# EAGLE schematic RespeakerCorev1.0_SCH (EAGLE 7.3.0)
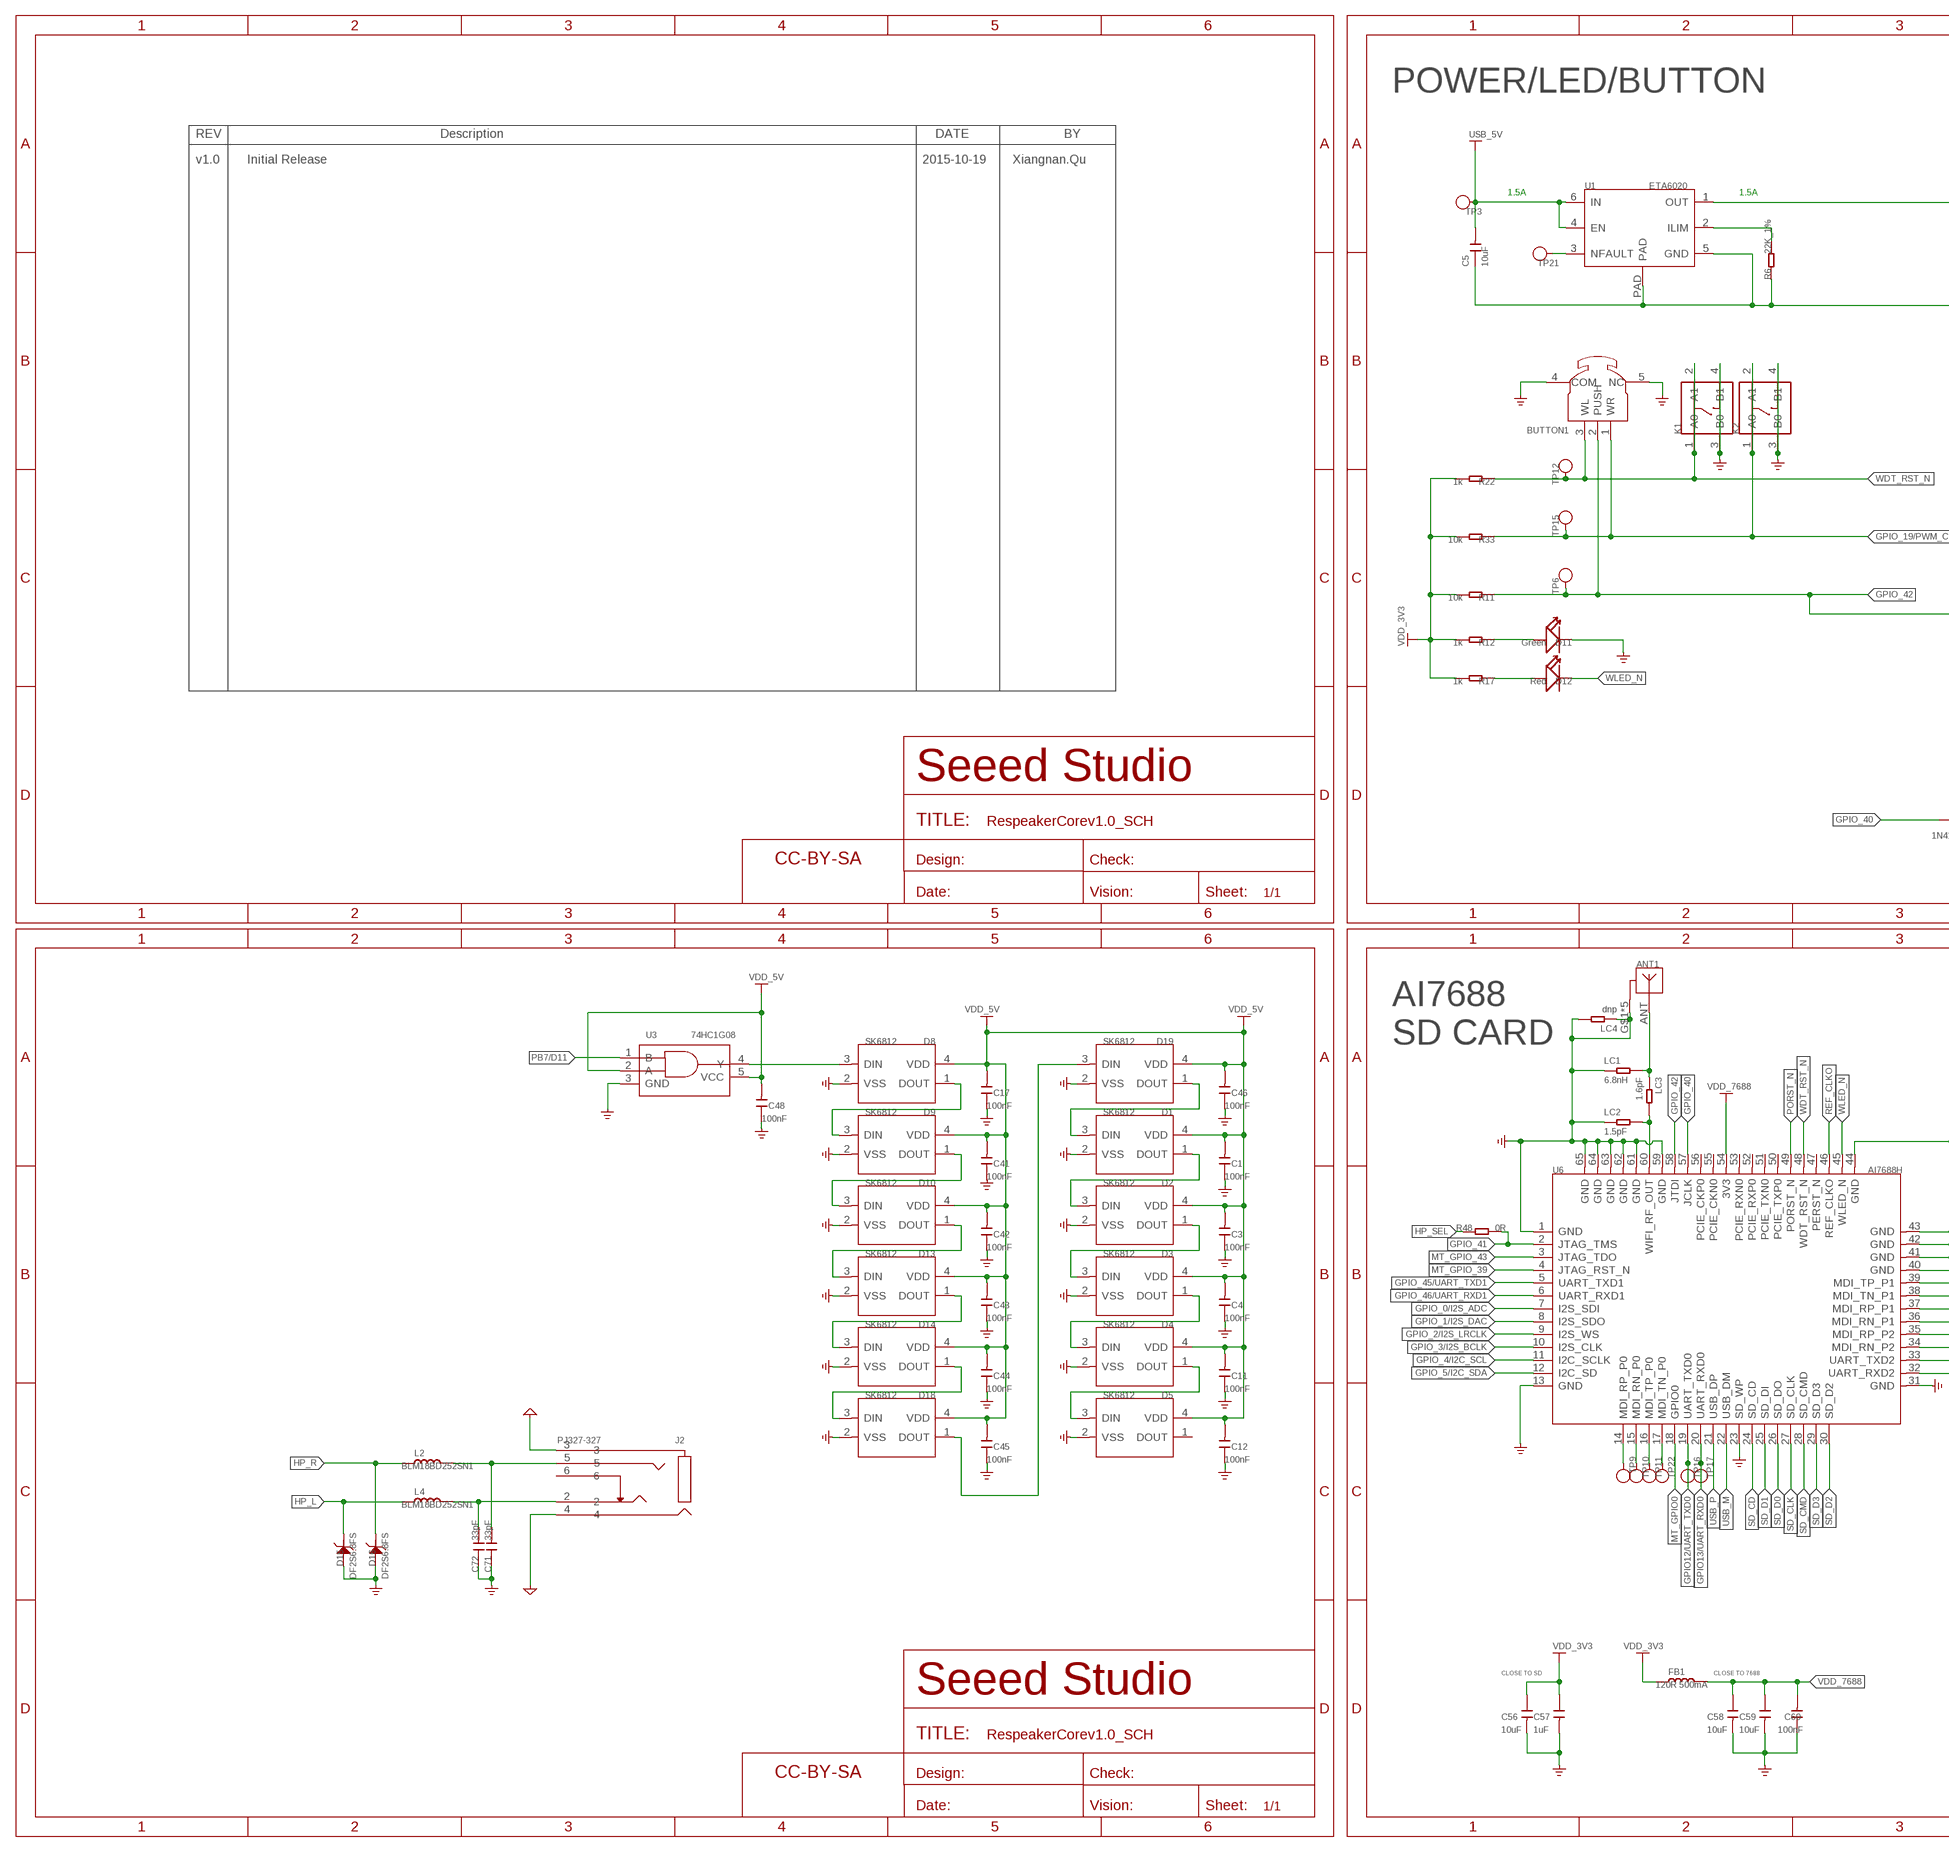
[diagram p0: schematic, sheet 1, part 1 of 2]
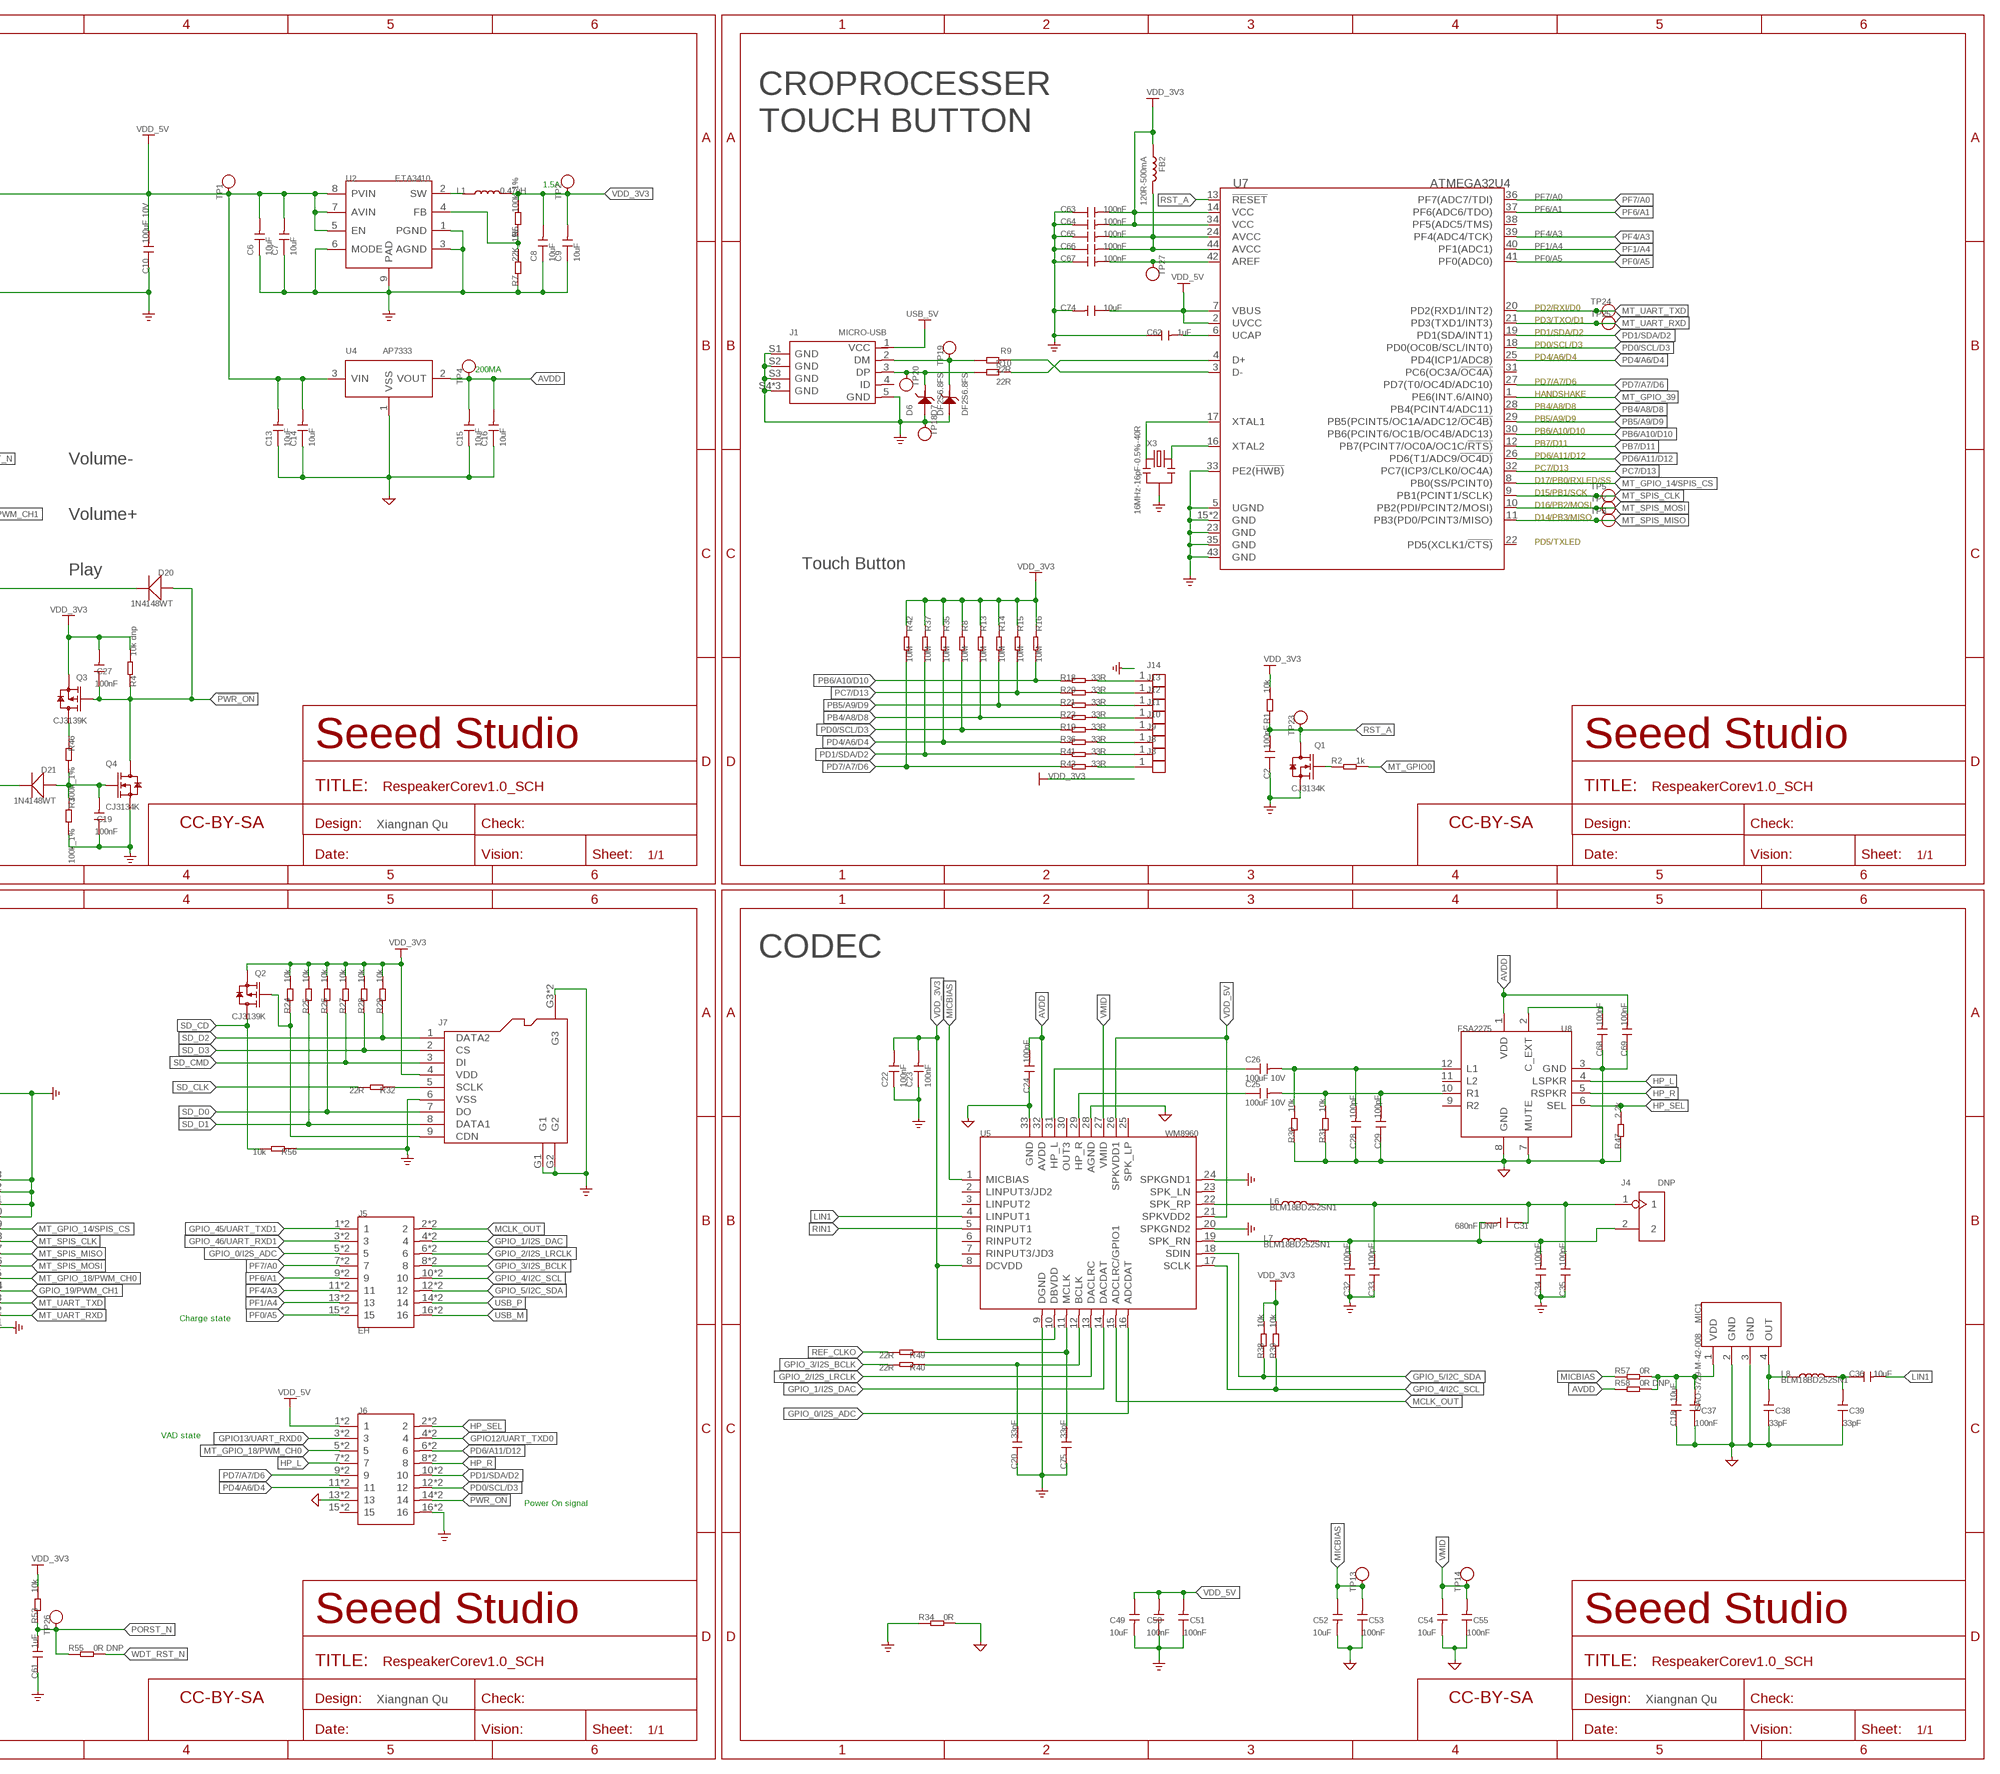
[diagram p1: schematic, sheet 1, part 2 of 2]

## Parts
ANT1  ANTENNA-ACA2012-BOTTOM  [ANT2P-SMD-3.5X1.4MM-BOTTOM]
BUTTON1  BUTTON3+2P  [BUTTON3+2P-SMD-11.8X11.8X2.5MM]
C1  100nF  CAP-0402  [C0402]
C2  100nF  CAP-0402  [C0402]
C3  100nF  CAP-0402  [C0402]
C4  100nF  CAP-0402  [C0402]
C5  10uF  CAP-0603  [C0603]
C6  10uF  CAP-0603  [C0603]
C7  10uF  CAP-0603  [C0603]
C8  10uF  CAP-0603  [C0603]
C9  10uF  CAP-0603  [C0603]
C10  100uF 10V  CAP-1206  [C1206]
C11  100nF  CAP-0402  [C0402]
C12  100nF  CAP-0402  [C0402]
C13  10uF  CAP-0603  [C0603]
C14  10uF  CAP-0603  [C0603]
C15  10uF  CAP-0603  [C0603]
C16  10uF  CAP-0603  [C0603]
C17  100nF  CAP-0402  [C0402]
C18  10uF  CAP-0603  [C0603]
C19  100nF  CAP-0402  [C0402]
C20  33pF  CAP-0402  [C0402]
C22  100nF  CAP-0402  [C0402]
C23  100nF  CAP-0402  [C0402]
C24  100nF  CAP-0402  [C0402]
C25  100uF 10V  CAP-1206  [C1206]
C26  100uF 10V  CAP-1206  [C1206]
C27  100nF  CAP-0402  [C0402]
C28  100pF  CAP-0402  [C0402]
C29  100pF  CAP-0402  [C0402]
C31  680nF DNP  CAP-0402  [C0402]
C32  100pF  CAP-0402  [C0402]
C33  100pF  CAP-0402  [C0402]
C34  100pF  CAP-0402  [C0402]
C35  100pF  CAP-0402  [C0402]
C36  10uF  CAP-0603  [C0603]
C37  100nF  CAP-0402  [C0402]
C38  33pF  CAP-0402  [C0402]
C39  33pF  CAP-0402  [C0402]
C41  100nF  CAP-0402  [C0402]
C42  100nF  CAP-0402  [C0402]
C43  100nF  CAP-0402  [C0402]
C44  100nF  CAP-0402  [C0402]
C45  100nF  CAP-0402  [C0402]
C46  100nF  CAP-0402  [C0402]
C48  100nF  CAP-0402  [C0402]
C49  10uF  CAP-0603  [C0603]
C50  100nF  CAP-0402  [C0402]
C51  100nF  CAP-0402  [C0402]
C52  10uF  CAP-0603  [C0603]
C53  100nF  CAP-0402  [C0402]
C54  10uF  CAP-0603  [C0603]
C55  100nF  CAP-0402  [C0402]
C56  10uF  CAP-0603  [C0603]
C57  1uF  CAP-0402  [C0402]
C58  10uF  CAP-0603  [C0603]
C59  10uF  CAP-0603  [C0603]
C60  100nF  CAP-0402  [C0402]
C61  1uF  CAP-0402  [C0402]
C62  1uF  CAP-0402  [C0402]
C63  100nF  CAP-0402  [C0402]
C64  100nF  CAP-0402  [C0402]
C65  100nF  CAP-0402  [C0402]
C66  100nF  CAP-0402  [C0402]
C67  100nF  CAP-0402  [C0402]
C68  100nF  CAP-0402  [C0402]
C69  100nF  CAP-0402  [C0402]
C71  33pF  CAP-0402  [C0402]
C72  33pF  CAP-0402  [C0402]
C74  10uF  CAP-0603  [C0603]
C75  33pF  CAP-0402  [C0402]
D1  SK6812  LED-RGB-4P-SK68122  [LED4-SMD-3.5X3.7MM]
D2  SK6812  LED-RGB-4P-SK68122  [LED4-SMD-3.5X3.7MM]
D3  SK6812  LED-RGB-4P-SK68122  [LED4-SMD-3.5X3.7MM]
D4  SK6812  LED-RGB-4P-SK68122  [LED4-SMD-3.5X3.7MM]
D5  SK6812  LED-RGB-4P-SK68122  [LED4-SMD-3.5X3.7MM]
D6  DF2S6.8FS  D-ESD-2P'DF2S6.8FS'  [SOD-923]
D7  DF2S6.8FS  D-ESD-2P'DF2S6.8FS'  [SOD-923]
D8  SK6812  LED-RGB-4P-SK68122  [LED4-SMD-3.5X3.7MM]
D9  SK6812  LED-RGB-4P-SK68122  [LED4-SMD-3.5X3.7MM]
D10  SK6812  LED-RGB-4P-SK68122  [LED4-SMD-3.5X3.7MM]
D11  Green  LED'RIGHT'  [LED-SIDE-VIEW-0603-RIGHT]
D12  Red  LED'RIGHT'  [LED-SIDE-VIEW-0603-RIGHT]
D13  SK6812  LED-RGB-4P-SK68122  [LED4-SMD-3.5X3.7MM]
D14  SK6812  LED-RGB-4P-SK68122  [LED4-SMD-3.5X3.7MM]
D15  DF2S6.8FS  D-ESD-2P'DF2S6.8FS'  [SOD-923]
D16  DF2S6.8FS  D-ESD-2P'DF2S6.8FS'  [SOD-923]
D18  SK6812  LED-RGB-4P-SK68122  [LED4-SMD-3.5X3.7MM]
D19  SK6812  LED-RGB-4P-SK68122  [LED4-SMD-3.5X3.7MM]
D20  1N4148WT  DIODE'0603'  [SOD-523]
D21  1N4148WT  DIODE'0603'  [SOD-523]
FB1  120R 500mA  INDUCTOR/FERRITE-BEAD'0603'  [L0603]
FB2  120R-500mA  INDUCTOR/FERRITE-BEAD'0603'  [L0603]
FR1  SEEEDSTUDIO-OPEN-SCH-FRAME  [SEEEDSTUDIO-PCB-FRAME]
FR2  SEEEDSTUDIO-OPEN-SCH-FRAME  [SEEEDSTUDIO-PCB-FRAME]
FR3  SEEEDSTUDIO-OPEN-SCH-FRAME  [SEEEDSTUDIO-PCB-FRAME]
FR4  SEEEDSTUDIO-OPEN-SCH-FRAME  [SEEEDSTUDIO-PCB-FRAME]
FR5  SEEEDSTUDIO-OPEN-SCH-FRAME  [SEEEDSTUDIO-PCB-FRAME]
FR7  SEEEDSTUDIO-OPEN-SCH-FRAME  [SEEEDSTUDIO-PCB-FRAME]
J1  MICRO-USB  MICRO-USB5+4P'5+4P'  [MICRO-USB5+4P-SMD-0.65-B]
J2  PJ327-327  AUDIO-JACK-5P-PJ327-327  [AUDIO5P-14X5X4.4MM]
J3  HEADER-1P-3MM  [1P-DIP-6X4MM]
J4  DNP  HEADER-2P-65/35MIL  [H2-2.54]
J5  EH  HEADER-2X8P-SMD_DRILL-2.0  [H2X8-SMD_DRILL-2.0]
J6  HEADER-2X8P-SMD_DRILL-2.0  [H2X8-SMD_DRILL-2.0]
J7  MICRO-SD-CARD-HOLDER-9P'MICROSD-9P'  [MICRO-SD9+4P-SMD-16.1X14.5X1.85MM]
J8  HEADER-1P-3MM  [1P-DIP-6X4MM]
J9  HEADER-1P-3MM  [1P-DIP-6X4MM]
J10  HEADER-1P-3MM  [1P-DIP-6X4MM]
J11  HEADER-1P-3MM  [1P-DIP-6X4MM]
J12  HEADER-1P-3MM  [1P-DIP-6X4MM]
J13  HEADER-1P-3MM  [1P-DIP-6X4MM]
J14  HEADER-1P-3MM  [1P-DIP-6X4MM]
K1  BUTTON-4P-4.5X3.2  [SW4P-SMD-4.5X3.2X2.5MM]
K2  BUTTON-4P-4.5X3.2  [SW4P-SMD-4.5X3.2X2.5MM]
L1  0.47uH  L-MPM201610SR33_T  [L201610]
L2  BLM18BD252SN1  INDUCTOR/FERRITE-BEAD'0603'  [L0603]
L4  BLM18BD252SN1  INDUCTOR/FERRITE-BEAD'0603'  [L0603]
L6  BLM18BD252SN1  INDUCTOR/FERRITE-BEAD'0603'  [L0603]
L7  BLM18BD252SN1  INDUCTOR/FERRITE-BEAD'0603'  [L0603]
L8  BLM18BD252SN1  INDUCTOR/FERRITE-BEAD'0603'  [L0603]
LC1  6.8nH  RES-0402  [R0402]
LC2  1.5pF  RES-0402  [R0402]
LC3  1.6pF  RES-0402  [R0402]
LC4  dnp  RES-0402  [R0402]
MIC1  SAO-3729-M-42-008  MIC-MSM421A3729H8-C  [MIC4-SMD-3.76X2.95MM]
Q1  CJ3134K  MOSFET-N-CJ3134K  [SOT-723]
Q2  CJ3139K  MOSFET-P-CJ3139K  [SOT-723]
Q3  CJ3139K  MOSFET-P-CJ3139K  [SOT-723]
Q4  CJ3134K  MOSFET-N-CJ3134K  [SOT-723]
R1  10k  RES-0402  [R0402]
R2  1k  RES-0402  [R0402]
R3  100k_1%  RES-0402  [R0402]
R4  10k dnp  RES-0402  [R0402]
R5  100k_1%  RES-0402  [R0402]
R6  22K_1%  RES-0402  [R0402]
R7  22K_1%  RES-0402  [R0402]
R8  10M  RES-0402  [R0402]
R9  22R  RES-0402  [R0402]
R10  22R  RES-0402  [R0402]
R11  10k  RES-0402  [R0402]
R12  1k  RES-0402  [R0402]
R13  10M  RES-0402  [R0402]
R14  10M  RES-0402  [R0402]
R15  10M  RES-0402  [R0402]
R16  10M  RES-0402  [R0402]
R17  1k  RES-0402  [R0402]
R18  33R  RES-0402  [R0402]
R19  33R  RES-0402  [R0402]
R20  33R  RES-0402  [R0402]
R21  33R  RES-0402  [R0402]
R22  1k  RES-0402  [R0402]
R23  33R  RES-0402  [R0402]
R24  10k  RES-0402  [R0402]
R25  10k  RES-0402  [R0402]
R26  10k  RES-0402  [R0402]
R27  10k  RES-0402  [R0402]
R28  10k  RES-0402  [R0402]
R29  10k  RES-0402  [R0402]
R30  10k  RES-0402  [R0402]
R31  10k  RES-0402  [R0402]
R32  22R  RES-0402  [R0402]
R33  10k  RES-0402  [R0402]
R34  0R  RES-0402  [R0402]
R35  10M  RES-0402  [R0402]
R36  33R  RES-0402  [R0402]
R37  10M  RES-0402  [R0402]
R38  10k  RES-0402  [R0402]
R39  10k  RES-0402  [R0402]
R40  22R  RES-0402  [R0402]
R41  33R  RES-0402  [R0402]
R42  10M  RES-0402  [R0402]
R43  33R  RES-0402  [R0402]
R46  100k_1%  RES-0402  [R0402]
R47  2.2k  RES-0402  [R0402]
R48  0R  RES-0402  [R0402]
R49  22R  RES-0402  [R0402]
R53  10k  RES-0402  [R0402]
R55  0R DNP  RES-0402  [R0402]
R56  10k  RES-0402  [R0402]
R57  0R  RES-0402  [R0402]
R58  0R DNP  RES-0402  [R0402]
TP1  TEST-POINT'4545'  [TP-D45MIL]
TP2  TEST-POINT'4545'  [TP-D45MIL]
TP3  TEST-POINT'4545'  [TP-D45MIL]
TP4  TEST-POINT'4545'  [TP-D45MIL]
TP5  TEST-POINT'4545'  [TP-D45MIL]
TP6  TEST-POINT'4545'  [TP-D45MIL]
TP7  TEST-POINT'4545'  [TP-D45MIL]
TP8  TEST-POINT'4545'  [TP-D45MIL]
TP9  TEST-POINT'4080'  [TP-80X40MIL]
TP10  TEST-POINT'4080'  [TP-80X40MIL]
TP11  TEST-POINT'4080'  [TP-80X40MIL]
TP12  TEST-POINT'4545'  [TP-D45MIL]
TP13  TEST-POINT'4545'  [TP-D45MIL]
TP14  TEST-POINT'4545'  [TP-D45MIL]
TP15  TEST-POINT'4545'  [TP-D45MIL]
TP16  TEST-POINT'4545'  [TP-D45MIL]
TP17  TEST-POINT'4545'  [TP-D45MIL]
TP18  TEST-POINT'4545'  [TP-D45MIL]
TP19  TEST-POINT'4545'  [TP-D45MIL]
TP20  TEST-POINT'4545'  [TP-D45MIL]
TP21  TEST-POINT'4545'  [TP-D45MIL]
TP22  TEST-POINT'4080'  [TP-80X40MIL]
TP23  TEST-POINT'4545'  [TP-D45MIL]
TP24  TEST-POINT'4545'  [TP-D45MIL]
TP25  TEST-POINT'4545'  [TP-D45MIL]
TP26  TEST-POINT'4545'  [TP-D45MIL]
TP27  TEST-POINT'4545'  [TP-D45MIL]
U1  ETA6020  PMIC-ETA6020D2G-T_UDFN6  [DFN6G-0.65-2X2MM]
U2  ETA3410  CONVERTER-ETA3410  [DFN8G-0.5-2X2MM]
U3  74HC1G08  LOGIC-74HC1G08'GW'  [SOT-353]
U4  AP7333  PMIC-XC6206PMR  [SOT-23]
U5  WM8960  AMPLIFIER-WM8960  [QFN32G-0.5-5X5MM]
U6  AI7688H  MOUDLE-IOT-AI7688H  [LGA65-1.7-24X32X1.8MM]
U7  ATMEGA32U4  MCU-ATMEGA32U4-MUR  [VQFN-44]
U8  FSA2275  SWITCH-ANALOG-FSA2275  [LEAD12P-SMD-0.4-1.8X1.8X0.5MM]
X3  16MHz-16pF-0.5%-40R  CRYSTAL-RESONATOR'SMD'  [RESONATOR3-SMD-3.6X1.3X0.8MM]

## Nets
!PWR_ON: C27.1 D20.+ J6.14 J6.P$14 Q3.1(G) Q4.3(D) R4.1
AGND: C13.1 C14.1 C15.1 C16.1 C18.1 C24.1 C28.1 C29.1 C37.1 C38.1 C39.1 C52.2 C53.1 C54.2 C55.1 C68.1 C69.1 J2.3 J2.4 J6.13 J6.P$13 MIC1.2(GND) MIC1.3(GND) R30.1 R31.1 R34.2 R47.1 U4.1(VSS) U5.28(AGND) U5.33(GND) U8.3(GND) U8.7(MUTE) U8.8(GND) ; supply symbol labelled GND_SIGNAL
AVDD: C15.2 C16.2 C24.2 C69.2 R58.1 TP4.T U4.2(VOUT) U5.32(AVDD) U8.1(VDD)
GND: ANT1.G$1 ANT1.G$2 ANT1.G$4 ANT1.GND1 ANT1.GND2 BUTTON1.4(COM) BUTTON1.5(NC) C1.1 C2.1 C3.1 C4.1 C5.1 C6.1 C7.1 C8.1 C9.1 C10.1 C11.1 C12.1 C17.1 C19.1 C20.1 C22.1 C23.1 C32.1 C33.1 C34.1 C35.1 C41.1 C42.1 C43.1 C44.1 C45.1 C46.1 C48.1 C49.2 C50.1 C51.1 C56.2 C57.2 C58.2 C59.2 C60.1 C61.1 C62.1 C63.1 C64.1 C65.1 C66.1 C67.1 C71.1 C72.1 C74.2 C75.1 D1.2(VSS) D2.2(VSS) D3.2(VSS) D4.2(VSS) D5.2(VSS) D6.2 D7.2 D8.2(VSS) D9.2(VSS) D10.2(VSS) D11.2(-) D13.2(VSS) D14.2(VSS) D15.2 D16.2 D18.2(VSS) D19.2(VSS) J1.5(GND) J1.S1(GND) J1.S2(GND) J1.S3(GND) J1.S4(GND) J1.S5(GND) J1.S6(GND) J6.16 J6.P$16 J7.6(VSS) J7.G1 J7.G2 J7.G3 J7.G4(G3) K1.3(B0) K1.4(B1) K2.3(B0) K2.4(B1) LC1.1 LC2.1 LC4.1 LC4.2 Q1.2(S) Q4.2(S) R3.2 R6.1 R7.1 R34.1 R56.1 TP18.T U1.5(GND) U1.PAD U2.1(PGND) U2.3(AGND) U2.6(MODE) U2.9(PAD) U3.3(GND) U5.9(DGND) U5.20(SPKGND2) U5.24(SPKGND1) U6.1(GND) U6.13(GND) U6.23(SD_WP) U6.31(GND) U6.40(GND) U6.41(GND) U6.42(GND) U6.43(GND) U6.44(GND) U6.59(GND) U6.61(GND) U6.62(GND) U6.63(GND) U6.64(GND) U6.65(GND) U7.5(UGND) U7.15(GND) U7.23(GND) U7.33(PE2(!HWB)) U7.35(GND) U7.43(GND) U7.TAB(GND) X3.2 ; supply symbol labelled GND_POWER
GPIO12/UART_TXD0: J6.4 J6.P$4 TP16.T U6.19(UART_TXD0)
GPIO13/UART_RXD0: J6.3 J6.P$3 TP17.T U6.20(UART_RXD0)
GPIO_0/I2S_ADC: J5.5 J5.P$5 U5.16(ADCDAT) U6.7(I2S_SDI)
GPIO_1/I2S_DAC: J5.4 J5.P$4 U5.14(DACDAT) U6.8(I2S_SDO)
GPIO_2/I2S_LRCLK: J5.6 J5.P$6 U5.13(DACLRC) U6.9(I2S_WS)
GPIO_3/I2S_BCLK: J5.8 J5.P$8 R40.2 U6.10(I2S_CLK)
GPIO_4/I2C_SCL: J5.10 J5.P$10 R39.1 U5.17(SCLK) U6.11(I2C_SCLK)
GPIO_5/I2C_SDA: J5.12 J5.P$12 R38.1 U5.18(SDIN) U6.12(I2C_SD)
GPIO_19/PWM_CH1: BUTTON1.1(WR) K2.1(A0) K2.2(A1) R33.1 TP15.T U6.34(MDI_RN_P2)
GPIO_40: D21.- U6.57(JCLK)
GPIO_41: R48.1 U6.2(JTAG_TMS)
GPIO_42: BUTTON1.2(PUSH) D20.- R11.1 TP6.T U6.58(JTDI)
GPIO_45/UART_TXD1: J5.1 J5.P$1 U6.5(UART_TXD1)
GPIO_46/UART_RXD1: J5.3 J5.P$3 U6.6(UART_RXD1)
HP_L: D15.1 J6.7 J6.P$7 L4.1 U8.4(LSPKR)
HP_R: D16.1 J6.8 J6.P$8 L2.1 U8.5(RSPKR)
HP_SEL: J6.2 J6.P$2 R47.2 R48.2 U8.6(SEL)
LIN1: C36.2 U5.4(LINPUT1)
MCLK_OUT: J5.2 J5.P$2 U5.15(ADCLRC/GPIO1)
MIC_VDD: C18.2 C37.2 MIC1.1(VDD) R57.2 R58.2
MICBIAS: C52.1 C53.2 R57.1 TP13.T U5.1(MICBIAS)
MT_GPIO0: R2.2 U6.18(GPIO0)
MT_GPIO_14/SPIS_CS: U6.39(MDI_TP_P1) U7.8(PB0(SS/PCINT0))
MT_GPIO_18/PWM_CH0: J6.5 J6.P$5 U6.35(MDI_RP_P2)
MT_GPIO_39: U6.4(JTAG_RST_N) U7.1(PE6(INT.6/AIN0))
MT_GPIO_43: U6.3(JTAG_TDO)
MT_SPIS_CLK: TP5.T U6.38(MDI_TN_P1) U7.9(PB1(PCINT1/SCLK))
MT_SPIS_MISO: TP8.T U6.37(MDI_RP_P1) U7.11(PB3(PD0/PCINT3/MISO))
MT_SPIS_MOSI: TP7.T U6.36(MDI_RN_P1) U7.10(PB2(PDI/PCINT2/MOSI))
MT_UART_RXD: TP25.T U6.32(UART_RXD2) U7.21(PD3(TXD1/INT3))
MT_UART_TXD: TP24.T U6.33(UART_TXD2) U7.20(PD2(RXD1/INT2))
N$1: Q3.3(D) R46.1
N$2: LC2.2 LC3.2 U6.60(WIFI_RF_OUT)
N$3: D11.1(+) R12.1
N$4: C68.2 U8.2(C_EXT)
N$5: C75.2 R49.1 U5.11(MCLK)
N$6: C38.2 L8.1 MIC1.4(OUT)
N$7: D12.1(+) R17.1
N$8: R10.1 U7.4(D+)
N$9: J7.5(SCLK) R32.1
N$10: R9.1 U7.3(D-)
N$11: D9.1(DOUT) D10.3(DIN)
N$12: R6.2 U1.2(ILIM)
N$13: D1.3(DIN) D19.1(DOUT)
N$14: L6.1 U5.22(SPK_RP)
N$15: D7.1 J1.2(DM) R9.2 TP19.T
N$16: D6.1 J1.3(DP) R10.2 TP20.T
N$18: D10.1(DOUT) D13.3(DIN)
N$19: D8.1(DOUT) D9.3(DIN)
N$20: J13.1 R20.2
N$21: C19.2 D21.+ Q4.1(G) R3.1 R46.2
N$22: J14.1 R18.2
N$23: D13.1(DOUT) D14.3(DIN)
N$24: C36.1 C39.2 L8.2
N$25: D14.1(DOUT) D18.3(DIN)
N$26: C20.2 R40.1 U5.12(BCLK)
N$27: TP9.1(T) U6.14(MDI_RP_P0)
N$28: Q1.1(G) R2.1
N$29: L1.1 U2.2(SW)
N$30: D18.1(DOUT) D19.3(DIN)
N$31: J8.1 R41.2
N$32: R5.1 R7.2 U2.4(FB)
N$33: J12.1 R21.2
N$34: J11.1 R23.2
N$35: J3.1 R43.2
N$36: J9.1 R36.2
N$37: J10.1 R19.2
N$38: L7.1 U5.19(SPK_RN)
N$39: C31.1 C33.2 C35.2 J4.1 L6.2
N$40: C62.2 U7.6(UCAP)
N$41: C67.2 TP27.T U7.42(AREF)
N$42: D1.1(DOUT) D2.3(DIN)
N$43 [none3]: C65.2 C66.2 FB2.2 U7.24(AVCC) U7.44(AVCC)
N$44: D2.1(DOUT) D3.3(DIN)
N$45: D3.1(DOUT) D4.3(DIN)
N$46: D4.1(DOUT) D5.3(DIN)
N$47: C31.2 C32.2 C34.2 J4.2 L7.2
N$49: U7.17(XTAL1) X3.1
N$50: U7.16(XTAL2) X3.3
N$51: ANT1.ANT LC1.2 LC3.1
N$52: TP10.1(T) U6.15(MDI_RN_P0)
N$53: TP11.1(T) U6.16(MDI_TP_P0)
N$54: TP22.1(T) U6.17(MDI_TN_P0)
N$57: C26.2 C28.2 R30.2 U8.12(L1)
N$58: C25.1 U5.29(HP_R)
N$59: D8.3(DIN) U3.4(Y)
N$60: C26.1 U5.31(HP_L)
N$61: C25.2 C29.2 R31.2 U8.10(R1)
N$63: C72.2 J2.2 L4.2
N$64: C71.2 J2.5 L2.2
PB4/A8/D8: R13.1 R23.1 U7.28(PB4(PCINT4/ADC11))
PB5/A9/D9: R14.1 R21.1 U7.29(PB5(PCINT5/OC1A/ADC12/!OC4B))
PB6/A10/D10: R16.1 R18.1 U7.30(PB6(PCINT6/OC1B/OC4B/ADC13))
PB7/D11: U3.1(B) U7.12(PB7(PCINT7/OC0A/OC1C/!RTS))
PC7/D13: R15.1 R20.1 U7.32(PC7(ICP3/CLK0/OC4A))
PD0/SCL/D3: J6.12 J6.P$12 R8.1 R19.1 U7.18(PD0(OC0B/SCL/INT0))
PD1/SDA/D2: J6.10 J6.P$10 R37.1 R41.1 U7.19(PD1(SDA/INT1))
PD4/A6/D4: J6.11 J6.P$11 R35.1 R36.1 U7.25(PD4(ICP1/ADC8))
PD6/A11/D12: J6.6 J6.P$6 U7.26(PD6(T1/ADC9/!OC4D))
PD7/A7/D6: J6.9 J6.P$9 R42.1 R43.1 U7.27(PD7(T0/OC4D/ADC10))
PF0/A5: J5.15 J5.P$15 U7.41(PF0(ADC0))
PF1/A4: J5.13 J5.P$13 U7.40(PF1(ADC1))
PF4/A3: J5.11 J5.P$11 U7.39(PF4(ADC4/TCK))
PF6/A1: J5.9 J5.P$9 U7.37(PF6(ADC6/TDO))
PF7/A0: J5.7 J5.P$7 U7.36(PF7(ADC7/TDI))
PORST_N: C61.2 R53.1 R55.1 TP26.T U6.49(PORST_N)
PW_FAULT: TP21.T U1.3(NFAULT)
REF_CLKO: R49.2 U6.46(REF_CLKO)
RIN1: U5.5(RINPUT1)
RST_A: C2.2 Q1.3(D) R1.1 TP23.T U7.13(!RESET)
SD_CD: Q2.3(D) R56.2 U6.24(SD_CD)
SD_CLK: R32.2 U6.27(SD_CLK)
SD_CMD: J7.3(DI) R27.1 U6.28(SD_CMD)
SD_D0: J7.7(DO) R26.1 U6.26(SD_DO)
SD_D1: J7.8(DATA1) R25.1 U6.25(SD_DI)
SD_D2: J7.1(DATA2) R29.1 U6.30(SD_D2)
SD_D3: J7.2(CS) R28.1 U6.29(SD_D3)
SSSS: J7.9(CDN) Q2.1(G) R24.1
USB_5V: C5.2 J1.1(VCC) TP3.T U1.4(EN) U1.6(IN) ; supply symbol labelled POWER_BAR
USB_M: J5.16 J5.P$16 U6.22(USB_DM)
USB_P: J5.14 J5.P$14 U6.21(USB_DP)
VDD_3V3: C8.2 C9.2 C22.2 C23.2 C27.2 C56.1 C57.1 C63.2 C64.2 FB1.1 FB2.1 J7.4(VDD) L1.2 Q2.2(S) Q3.2(S) R1.2 R4.2 R5.2 R8.2 R11.2 R12.2 R13.2 R14.2 R15.2 R16.2 R17.2 R22.2 R24.2 R25.2 R26.2 R27.2 R28.2 R29.2 R33.2 R35.2 R37.2 R38.2 R39.2 R42.2 R53.2 TP2.T U5.8(DCVDD) U5.10(DBVDD) U7.14(VCC) U7.34(VCC) ; supply symbol labelled POWER_BAR
VDD_5V: C1.2 C3.2 C4.2 C6.2 C7.2 C10.2 C11.2 C12.2 C13.2 C14.2 C17.2 C41.2 C42.2 C43.2 C44.2 C45.2 C46.2 C48.2 C49.1 C50.2 C51.2 C74.1 D1.4(VDD) D2.4(VDD) D3.4(VDD) D4.4(VDD) D5.4(VDD) D8.4(VDD) D9.4(VDD) D10.4(VDD) D13.4(VDD) D14.4(VDD) D18.4(VDD) D19.4(VDD) J6.1 J6.P$1 TP1.T U1.1(OUT) U2.5(EN) U2.7(AVIN) U2.8(PVIN) U3.2(A) U3.5(VCC) U4.3(VIN) U5.21(SPKVDD2) U5.26(SPKVDD1) U7.2(UVCC) U7.7(VBUS) ; supply symbol labelled POWER_BAR
VDD_7688: C58.1 C59.1 C60.2 FB1.2 U6.54(3V3) ; supply symbol labelled POWER_BAR
VMID: C54.1 C55.2 TP14.T U5.27(VMID)
WDT_RST_N: BUTTON1.3(WL) K1.1(A0) K1.2(A1) R22.1 R55.2 TP12.T U6.48(WDT_RST_N)
WLED_N: D12.2(-) U6.45(WLED_N)
Unconnected: D5.1(DOUT) J1.4(ID) J2.6 J6.15 J6.P$15 U5.2(LINPUT3/JD2) U5.3(LINPUT2) U5.6(RINPUT2) U5.7(RINPUT3/JD3) U5.23(SPK_LN) U5.25(SPK_LP) U5.30(OUT3) U6.47(PERST_N) U6.50(PCIE_TXP0) U6.51(PCIE_TXN0) U6.52(PCIE_RXP0) U6.53(PCIE_RXN0) U6.55(PCIE_CKN0) U6.56(PCIE_CKP0) U7.22(PD5(XCLK1/!CTS)) U7.31(PC6(OC3A/!OC4A)) U7.38(PF5(ADC5/TMS)) U8.9(R2) U8.11(L2)

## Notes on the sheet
- POWER/LED/BUTTON
- CROPROCESSER
  TOUCH BUTTON
- v1.0 | Initial Release | 2015-10-19 | Xiangnan.Qu
- 1.5A | 1.5A | 1.5A
- PD2/RXI/D0
- PD3/TXO/D1
- PD1/SDA/D2
- PD0/SCL/D3
- PD4/A6/D4
- 200MA
- PD7/A7/D6
- HANDSHAKE
- PB4/A8/D8
- PB5/A9/D9
- PB6/A10/D10
- PB7/D11
- PD6/A11/D12
- Volume-
- PC7/D13
- D17/PB0/RXLED/SS
- D15/PB1/SCK
- D16/PB2/MOSI
- Volume+ | D14/PB3/MISO
- PD5/TXLED
- Touch Button
- Play
- Xiangnan Qu
- CODEC
- AI7688
  SD CARD
- Charge state
- VAD state
- Power On signal
- CLOSE TO SD | CLOSE TO 7688
- Xiangnan Qu | Xiangnan Qu

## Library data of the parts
ANT1 = Connector-new:ANTENNA-ACA2012
BUTTON1 = template:BUTTON3+2P
C1-C20 C22-C29 C31-C39 C41-C46 C48-C69 C71 C72 C74 C75 = Discrete-new:CAP: Ceramic Capacitors
D1-D5 D8-D10 D13 D14 D18 D19 = Discrete-new:LED-RGB-4P: 304990003
D6 D7 D15 D16 = Discrete-new:D-ESD-2P: SOD-923:304060009;SOD-123:304060001
D11 D12 = Discrete-new:LED
D20 D21 = Discrete-new:DIODE*
FB1 FB2 L2 L4 L6-L8 = Discrete-new:INDUCTOR/FERRITE-BEAD
FR1-FR5 FR7 = moudle-new:SEEEDSTUDIO-OPEN-SCH-FRAME
J1 = Connector-new:MICRO-USB5+4P: 5+4P-SMD-0.65-B:320010000;5+2P-SMD-0.65-AB:340032001
J2 = template:AUDIO-JACK-5P-PJ327
J3 J8-J14 = Connector-new:HEADER-1P
J4 = Connector-new:HEADER-2P
J5 J6 = Connector-new:HEADER-2X8P
J7 = Connector-new:MICRO-SD-CARD-HOLDER-9P: 320090000; SKU: 320090000
K1 K2 = Discrete-new:BUTTON-4P: SW4-6.0X6.0X5.0MM:311020024;SW4-8.0X8.0X9.0MM:311020028;SW4-SMD-6.0X6.0X5.0MM:311020004;SW4-SMD-3.35X3.35X1.5MM:311020030;SW4-SMD-5.2X5.2X2.5MM:311020046
L1 = Discrete-new:L
LC1-LC4 R1-R43 R46-R49 R53 R55-R58 = Discrete-new:RES
MIC1 = Connector-new:MIC-MSM421A3729H8-C
Q1 Q4 = Discrete-new:MOSFET-N
Q2 Q3 = Discrete-new:MOSFET-P
TP1-TP8 TP12-TP21 TP23-TP27 = Discrete-new:TEST-POINT; PARTNO: DNP
TP9-TP11 TP22 = Discrete-new:TEST-POINT
U1 = IC-new:PMIC-ETA6020D2G-T_U: 310990024
U2 = IC-new:CONVERTER-ETA3410: 3MHZ 2A High Step-Down Converter in DFN2x2-8L Package
U3 = IC-new:LOGIC-74HC1G08: 2-input AND gate
U4 = IC-new:PMIC-XC6206P: LOW ESR Cap.Compatible Positive Voltage Regulators
U5 = IC-new:AMPLIFIER-WM8960
U6 = moudle-new:MOUDLE-IOT-AI7688H
U7 = IC-new:MCU-ATMEGA32U4: TQFP-44:310010010;VQFN-44:310010016
U8 = template:SWITCH-ANALOG-FSA2275
X3 = Discrete-new:CRYSTAL-RESONATOR: Resonator Small SMD resonator. This is the itty bitty 10/20MHz resonators with built in caps. CSTCE10M0G55 and CSTCE20M0V53. Footprint has been reviewed closely but hasn't been tested yet.

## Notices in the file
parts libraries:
moudle-new: This work is licensed under the Creative Commons Attribution 4.0 International License.
To view a copy of this license,visit:
http://creativecommons.org/licenses/by-sa/4.0
moudle-new: CC-BY-SA
